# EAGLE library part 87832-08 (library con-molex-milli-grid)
HEADER
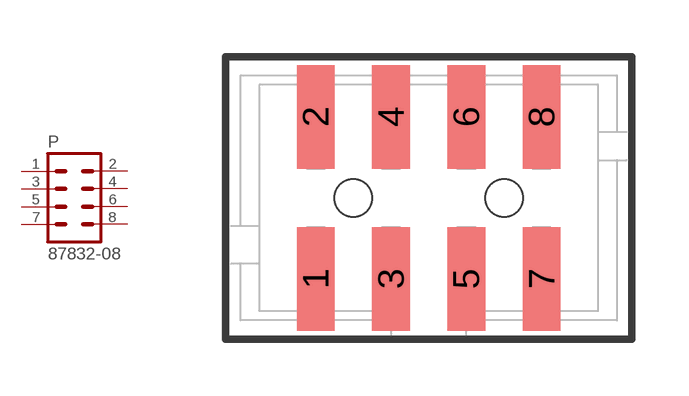
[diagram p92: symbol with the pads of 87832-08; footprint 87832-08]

Designator prefix P

## 87832-08  [87832-08]
1  1  pas
2  2  pas
3  3  pas
4  4  pas
5  5  pas
6  6  pas
7  7  pas
8  8  pas

## Footprint 87832-08 (pad centres in mm)
HEADER SMD Dual Row, Shrouded, Vertical
smd 1 x 2.75: 1 -3,-2.15; 2 -3,2.15; 3 -1,-2.15; 4 -1,2.15; 5 1,-2.15; 6 1,2.15; 7 3,-2.15; 8 3,2.15
hole 1 at -2,0
hole 1 at 2,0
